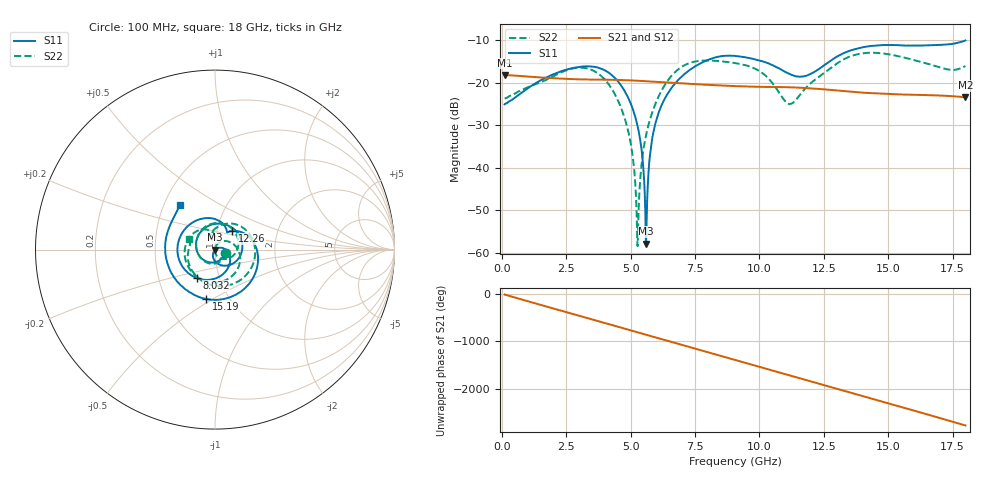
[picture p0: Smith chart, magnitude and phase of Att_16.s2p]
#  HZ  S  DB  R  50.00
! Rohde & Schwarz Vector Network Analyzer
! Rohde-Schwarz,ZNB40-4Port,1311601084101679,3.45
! Created: UTC 4/25/2025, 8:46:02 AM
! freq[Hz]  db:S11  ang:S11  db:S21  ang:S21  db:S12  ang:S12  db:S22  ang:S22
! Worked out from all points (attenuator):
!   1750 points, 100 MHz to 18 GHz, reference 50 ohm
!   highest |S21| = -18.12 dB at 100 MHz (marker M1); lowest = -23.4 dB at 18 GHz (marker M2)
!   lowest |S11| = -57.8 dB at 5.596 GHz (marker M3), VSWR 1.00, Z = 50.1 - j0.0706 ohm
!   |S11| at or under -10 dB: start of sweep to end of sweep
!   |S22| runs from -58.4 to -12.9 dB; largest |S21 - S12| = 0.00015
!   S11 on the Smith chart (normalised r, x): 100 MHz: 1.11, -0.04; 8.032 GHz: 0.78, -0.26; 12.26 GHz: 1.19, +0.25; 15.19 GHz: 0.78, -0.47; 18 GHz: 0.61, +0.34
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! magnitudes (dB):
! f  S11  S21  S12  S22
! 100 MHz  -25.0  -18.1  -18.1  -23.7
! 3.088 GHz  -16.2  -19.2  -19.2  -16.4
! 3.948 GHz  -16.9  -19.2  -19.2  -18.9
! 4.613 GHz  -20.5  -19.3  -19.3  -25.7
! 5.023 GHz  -25.2  -19.4  -19.4  -35.1
! 5.258 GHz  -30.0  -19.5  -19.5  -58.1
! 5.32 GHz  -31.7  -19.5  -19.5  -48.0
! 5.422 GHz  -35.8  -19.5  -19.5  -39.1
! 5.596 GHz  -57.8  -19.6  -19.6  -32.3
! 5.801 GHz  -34.4  -19.6  -19.6  -27.6
! 6.067 GHz  -27.3  -19.7  -19.7  -23.4
! 6.906 GHz  -18.9  -20.1  -20.1  -16.5
! 8.032 GHz  -14.5  -20.5  -20.5  -14.7
! 9.055 GHz  -13.6  -20.8  -20.8  -15.3
! 10.11 GHz  -14.9  -20.9  -20.9  -17.7
! 11.14 GHz  -17.8  -21.0  -21.0  -25.0
! 12.04 GHz  -17.7  -21.3  -21.3  -19.8
! 12.26 GHz  -16.9  -21.4  -21.4  -18.8
! 13.58 GHz  -12.3  -22.1  -22.1  -13.6
! 15.02 GHz  -11.1  -22.6  -22.6  -13.3
! 15.19 GHz  -11.1  -22.6  -22.6  -13.4
! 18 GHz  -10.0  -23.4  -23.4  -16.0
